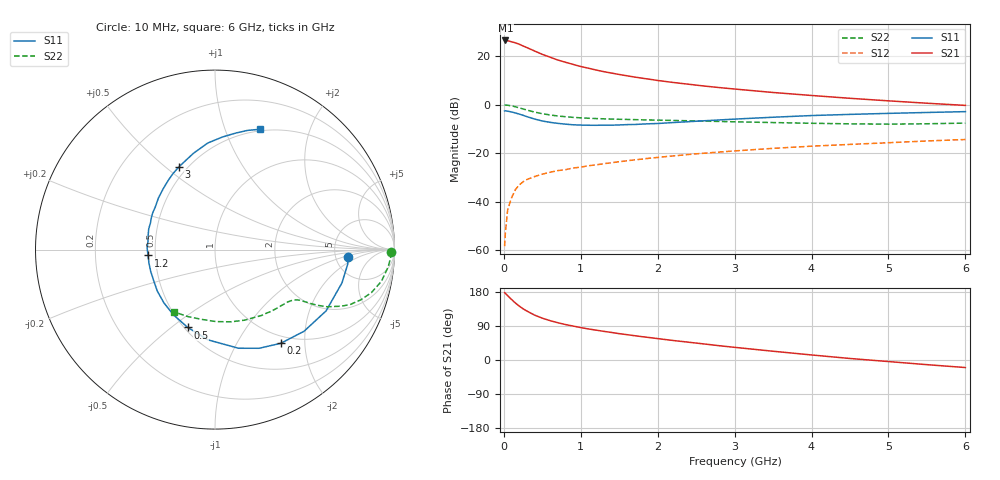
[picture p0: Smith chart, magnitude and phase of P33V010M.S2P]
! SIEMENS Small Signal Semiconductors
! BFP181
! Si NPN RF Bipolar Junction Transistor in SOT143
! VCE = 3 V  IC = 10 mA
! Common Emitter S-Parameters:  March  1996
# GHz  S  MA  R  50
!  f  S11  S21  S12  S22
! GHz  MAG  ANG  MAG  ANG  MAG  ANG  MAG  ANG
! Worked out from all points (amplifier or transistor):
!   36 points, 10 MHz to 6 GHz, reference 50 ohm
!   highest |S21| = 26.5 dB at 20 MHz (marker M1)
!   |S21| within 3 dB of that: start of sweep to 304.2 MHz
!   unconditionally stable (mu >= 1): 1.115 GHz to end of sweep
!   at 250 MHz: K = 0.35, MSG = 28.0 dB, |S12| = -31.8 dB
!   at 1.4 GHz: K = 1.09, MAG = 16.7 dB, |S12| = -24.0 dB
!   at 6 GHz: K = 1.01, MAG = 6.4 dB, |S12| = -14.4 dB
!   S11 on the Smith chart (normalised r, x): 10 MHz: 6.47, -1.14; 200 MHz: 0.88, -1.55; 500 MHz: 0.52, -0.57; 1.2 GHz: 0.46, -0.03; 3 GHz: 0.45, +0.56; 6 GHz: 0.48, +1.33
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0.01  0.7394 -3.1  20.96 177.7  0.0012 80.7  0.98 -0.9
0.02  0.744 -6.2  21.1 176.0  0.0023 87.6  0.981 -2.1
0.05  0.7313 -14.7  20.81 169.6  0.0068 84.4  0.9702 -5.6
0.1  0.7068 -28.9  19.82 159.8  0.0119 75.6  0.944 -10.8
0.15  0.6732 -42.5  18.86 150.4  0.0176 69.8  0.9034 -15.4
0.2  0.6379 -54.9  17.63 142.3  0.022 65.5  0.8593 -19.0
0.25  0.6023 -65.9  16.22 135.1  0.0256 61.1  0.8144 -22.0
0.3  0.565 -76.6  15.04 129.2  0.0285 58.4  0.7721 -24.1
0.4  0.5043 -94.5  12.78 118.4  0.0328 53.8  0.7017 -27.0
0.5  0.4596 -109.3  10.9 110.4  0.0368 50.5  0.6502 -28.5
0.6  0.4309 -122.5  9.545 103.9  0.0402 49.6  0.6122 -29.4
0.7  0.4112 -133.8  8.339 98.4  0.0434 49.1  0.5833 -30.0
0.9  0.3839 -152.2  6.765 89.6  0.0491 48.7  0.5459 -31.0
1.1  0.3755 -168.3  5.639 81.9  0.0546 48.8  0.5236 -32.4
1.2  0.3746 -175.0  5.177 78.8  0.0573 48.7  0.5159 -33.2
1.7  0.3891 157.5  3.707 64.1  0.0725 48.5  0.4902 -38.3
2.2  0.4266 137.6  2.869 51.5  0.0873 46.5  0.4714 -44.8
3  0.503 113.6  2.098 33.4  0.1108 41.6  0.4417 -57.7
3.5  0.5494 102.7  1.781 23.1  0.1253 38.5  0.4266 -67.1
4.5  0.6288 86.2  1.351 4.0  0.1512 30.8  0.4013 -89.0
5.5  0.6886 74.7  1.069 -12.3  0.1779 23.8  0.4028 -112.0
6  0.717 69.3  0.964 -19.9  0.1907 19.6  0.4158 -123.7
